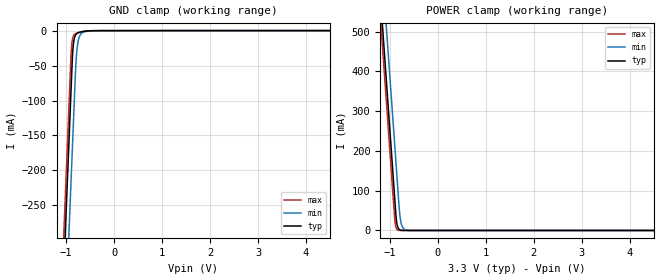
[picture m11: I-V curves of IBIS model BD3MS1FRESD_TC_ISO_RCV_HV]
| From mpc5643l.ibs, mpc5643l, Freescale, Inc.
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| *** New cell (Generated with 5.14beta1 (Sep 20 2010 13:23:23))
[Model]   BD3MS1FRESD_TC_ISO_RCV_HV
Model_type Input
Polarity   Non-Inverting
Enable   Active-Low
| CAP_THRESHOLD on pad pad is "CMOS" :
| Rising=10.0% of VDDE1   Falling=90.0% of VDDE1
| C_comp min and max val. don't necessarily correlate with the min and max pvt
| but are the smallest and greatest pad capacitance found.
| var   typ   min   max
C_comp   2.74556pF  2.55925pF  2.97762pF
Vinl = 1.05V | Dummy value overriden by next lines
Vinh = 2.34V | Dummy value overriden by next lines
[Model Spec]
| TIME_THRESHOLD on pin reset is "CORE" :
| Rising=40.0% of VDDE1   Falling=60.0% of VDDE1
Vinl 1.33350V 1.21150V 1.44350V
Vinh 1.90350V 1.71650V 2.07050V
| variable   typ   min   max
[Temperature Range] 25.0 150.0 -40.0
| variable   typ   min   max
[Voltage Range] 3.3V 3.0V 3.6V
| variable   typ   min   max
[POWER Clamp Reference] 3.3V 3.0V 3.6V
| variable   typ   min   max
[GND Clamp Reference] 0V 0V 0V
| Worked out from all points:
|   GND clamp passes 1 mA (typ) near -0.62 V on its own axis
|   POWER clamp passes 1 mA (typ) near -0.78 V on its own axis
[POWER Clamp]
-3.3V     4.162A     4.297A     4.11A
-1.21V    609.4mA    743.8mA    556.6mA
-1.14V    490.4mA    624.8mA    437.6mA
-1.07V    371.4mA    505.8mA    318.6mA
-900mV    82.42mA    216.8mA    29.59mA
-870mV    32.81mA    165.8mA    6.648mA
-830mV    6.917mA    97.75mA    908uA
-800mV    2.152mA    48.46mA    204uA
-760mV    453.6uA    16.18mA    27.88uA
-710mV    64.78uA    4.107mA    2.313uA
-630mV    2.867uA    457.8uA    31.47nA
6.6V      0A         0A         0A
[GND Clamp]
-3.3V     -4.17A     -4.3A      -4.118A
-1.08V    -395.6mA   -526mA     -344.3mA
-900mV    -89.65mA   -220mA     -38.3mA
-880mV    -55.65mA   -186mA     -17.69mA
-860mV    -28.03mA   -152mA     -9.747mA
-830mV    -11.47mA   -101mA     -5.624mA
-800mV    -5.903mA   -51.81mA   -4.156mA
-790mV    -4.99mA    -40.2mA    -3.843mA
-760mV    -3.4mA     -19.31mA   -3.086mA
-710mV    -2.181mA   -6.608mA   -2.083mA
-490mV    -176.6uA   -458.7uA   -113.3uA
6.6V      59.15uA    29.76uA    102.3uA
